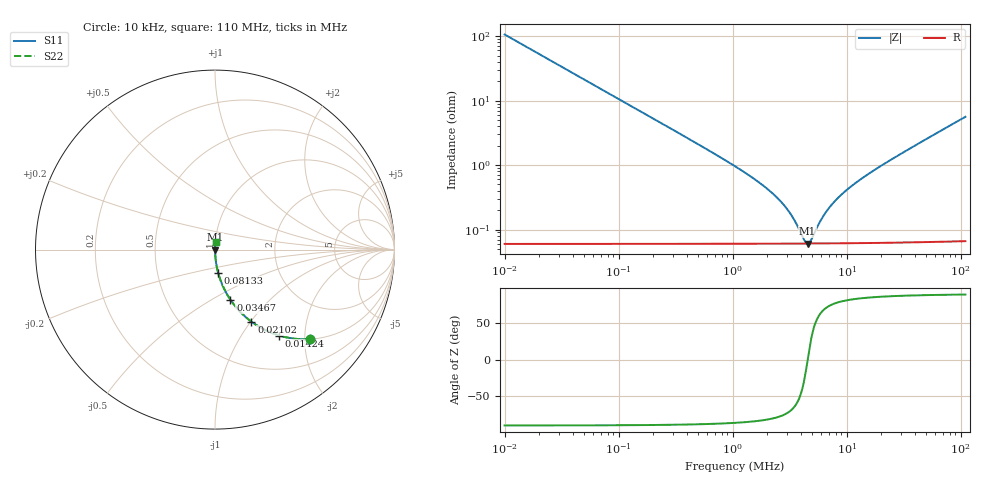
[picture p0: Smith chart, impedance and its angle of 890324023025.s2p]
! Touchstone file was created by TriD Version 2018.1.0 (64-bit) (07.02.2018)
! (C) EMCoS 1999-2018
! Project : CAP\TRID_890324023025_3mm_ports_Task 1\Task 1.in
! Date  : 2018-06-12  13:05:47
# HZ S RI R  50.00
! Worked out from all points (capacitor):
!   503 points, 10 kHz to 110 MHz, reference 50 ohm
!   read as one part in series: C = 150 nF near 10.39 kHz
!   lowest |Z| = 60.7 mohm at 4.539 MHz (marker M1)
!   series resonance near 4.549 MHz, so ESL is about 8.2 nH
!   S11 on the Smith chart (normalised r, x): 10 kHz: 1.00, -2.12; 14.24 kHz: 1.00, -1.49; 21.02 kHz: 1.00, -1.01; 34.67 kHz: 1.00, -0.61; 81.33 kHz: 1.00, -0.26; 110 MHz: 1.00, +0.08
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10000  0.5296 -0.4988  0.4704 0.4988  0.4704 0.4988  0.5296 -0.4988
14244  0.357 -0.4787  0.643 0.4787  0.643 0.4787  0.357 -0.4787
21022  0.2033 -0.4019  0.7967 0.4019  0.7967 0.4019  0.2033 -0.4019
34674  0.0861 -0.2795  0.9139 0.2795  0.9139 0.2795  0.0861 -0.2795
47516  0.048 -0.2124  0.952 0.2124  0.952 0.2124  0.048 -0.2124
81333  0.0173 -0.1281  0.9827 0.1281  0.9827 0.1281  0.0173 -0.1281
225410  0.0028 -0.0468  0.9972 0.0468  0.9972 0.0468  0.0028 -0.0468
1049700  0.000693 -0.00969  0.9993 0.00942  0.9993 0.00942  0.000693 -0.00969
1830300  0.000627 -0.00509  0.9994 0.00461  0.9994 0.00461  0.000627 -0.00509
2701200  0.000611 -0.00289  0.9994 0.00218  0.9994 0.00218  0.000611 -0.00289
3566900  0.000607 -0.00161  0.9994 0.000676  0.9994 0.000676  0.000607 -0.00161
3986500  0.000606 -0.00114  0.9994 9.42e-05  0.9994 9.42e-05  0.000606 -0.00114
4538700  0.000606 -0.000604  0.9994 -0.000584  0.9994 -0.000584  0.000606 -0.000604
4979500  0.000607 -0.00023  0.9994 -0.00107  0.9994 -0.00107  0.000607 -0.00023
5264200  0.000607 -6.18e-06  0.9994 -0.00137  0.9994 -0.00137  0.000607 -6.17e-06
5565200  0.000608 0.000217  0.9994 -0.00167  0.9994 -0.00167  0.000608 0.000217
7626300  0.000615 0.00152  0.9994 -0.00351  0.9994 -0.00351  0.000615 0.00152
8682700  0.00062 0.00209  0.9994 -0.00436  0.9994 -0.00436  0.00062 0.00209
1.0259e7  0.000628 0.00287  0.9994 -0.00556  0.9994 -0.00556  0.000628 0.00287
1.4589e7  0.000658 0.00482  0.9993 -0.00864  0.9993 -0.00864  0.000658 0.00482
2.3622e7  0.000749 0.00853  0.9992 -0.0147  0.9992 -0.0147  0.000749 0.00853
1.1e8  0.00359 0.0415  0.996 -0.0703  0.996 -0.0703  0.00358 0.0415
